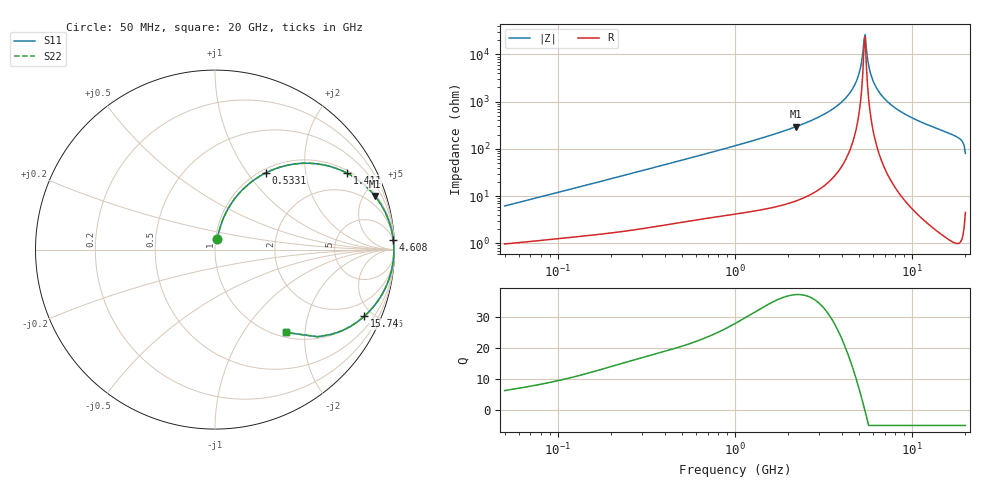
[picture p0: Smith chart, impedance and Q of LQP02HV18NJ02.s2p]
!Murata Part Number: LQP02HV18NJ02
!These Parameters are Measured in Series Mode Connection
!  o--[Z]--o
!Port1  Port2
!  o-------o
!Freq. Start=50[MHz] Stop=20[GHz], 401[Steps]
# Hz S RI R 50
!Freq.(Hz) S11(Real) S11(Imag) S21(Real) S21(Imag) S12(Real) S12(Imag) S22(Real) S22(Imag)
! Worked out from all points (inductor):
!   401 points, 50 MHz to 20 GHz, reference 50 ohm
!   read as one part in series: L = 19.2 nH near 51.52 MHz
!   highest Q = 37.3 at 2.212 GHz (marker M1), where L = 21.2 nH
!   self-resonance near 5.353 GHz
!   S11 on the Smith chart (normalised r, x): 50 MHz: 1.02, +0.12; 533.1 MHz: 1.06, +1.22; 1.411 GHz: 1.10, +3.38; 4.608 GHz: 4, +37; 15.74 GHz: 1.03, -4.46; 20 GHz: 1.09, -1.60
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5e7  0.0132 0.0596  0.9868 -0.0596  0.9868 -0.0596  0.0132 0.0596
1.364002e8  0.0381 0.1523  0.9619 -0.1523  0.9619 -0.1523  0.0381 0.1523
3.721004e8  0.1687 0.3484  0.8313 -0.3484  0.8313 -0.3484  0.1687 0.3484
5.330693e8  0.282 0.4269  0.718 -0.4269  0.718 -0.4269  0.282 0.4269
1e9  0.5716 0.4773  0.4284 -0.4773  0.4284 -0.4773  0.5716 0.4773
1.411297e9  0.7344 0.4268  0.2656 -0.4268  0.2656 -0.4268  0.7344 0.4268
2.211938e9  0.8907 0.2989  0.1093 -0.2989  0.1093 -0.2989  0.8907 0.2989
2.728004e9  0.9372 0.2291  0.0628 -0.2291  0.0628 -0.2291  0.9372 0.2291
3.792786e9  0.9812 0.118  0.0188 -0.118  0.0188 -0.118  0.9812 0.118
4.608136e9  0.9933 0.0531  0.0067 -0.0531  0.0067 -0.0531  0.9933 0.0531
4.966507e9  0.9956 0.0282  0.00444 -0.0282  0.00444 -0.0282  0.9956 0.0282
5.117541e9  0.9961 0.0183  0.0039 -0.0183  0.0039 -0.0183  0.9961 0.0183
5.273168e9  0.9964 0.00835  0.00356 -0.00835  0.00356 -0.00835  0.9964 0.00835
5.433528e9  0.9966 -0.00159  0.00342 0.00159  0.00342 0.00159  0.9966 -0.00159
5.515528e9  0.9966 -0.00657  0.00342 0.00657  0.00342 0.00657  0.9966 -0.00657
5.769027e9  0.9963 -0.0215  0.00375 0.0215  0.00375 0.0215  0.9963 -0.0215
6.125241e9  0.9951 -0.0415  0.0049 0.0415  0.0049 0.0415  0.9951 -0.0415
7.442007e9  0.9855 -0.107  0.0145 0.107  0.0145 0.107  0.9855 -0.107
9.892087e9  0.9531 -0.2054  0.0469 0.2054  0.0469 0.2054  0.9531 -0.2054
1.573793e10  0.8313 -0.3717  0.1687 0.3717  0.1687 0.3717  0.8313 -0.3717
1.855685e10  0.7289 -0.4414  0.2711 0.4414  0.2711 0.4414  0.7289 -0.4414
2e10  0.3956 -0.4617  0.6044 0.4617  0.6044 0.4617  0.3956 -0.4617
